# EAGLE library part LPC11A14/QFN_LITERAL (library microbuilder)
LPC11A14/QFN33 - 50MHz ARM Cortex M0 with 32kb Flash, 8kb SRAM, 10-bit ADC and DAC, Temperature Sensor, Analog Comparator, and 4kb EEPROM Temp Range: -40°C - 85°C VDD: 2.6-3.6V
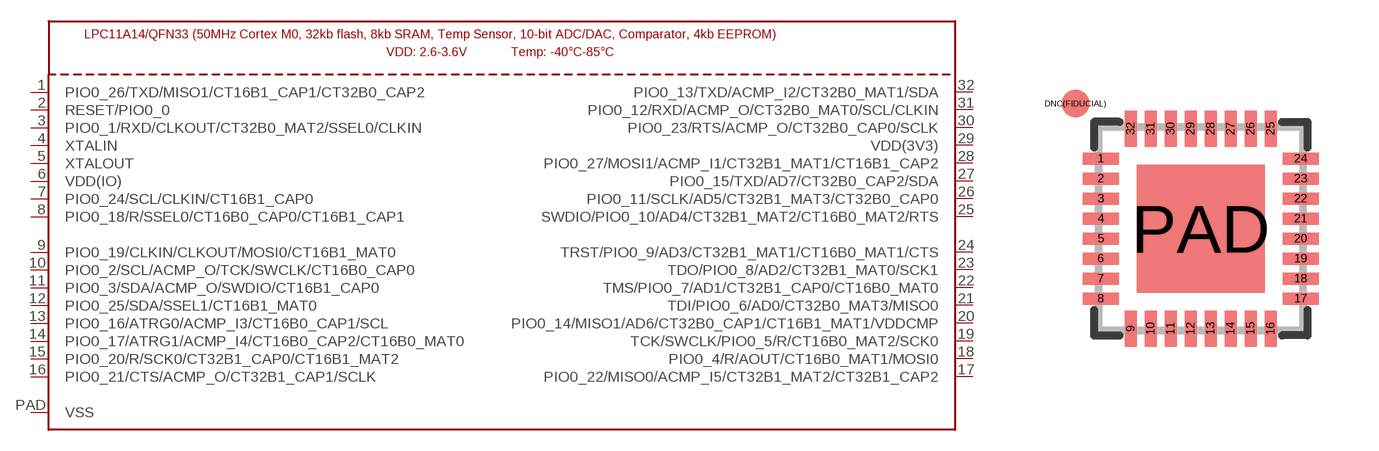
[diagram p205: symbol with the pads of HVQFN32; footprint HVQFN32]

Designator prefix U

## LPC11A14/QFN_LITERAL  [HVQFN32]
1  PIO0_26/TXD/MISO1/CT16B1_CAP1/CT32B0_CAP2
2  RESET/PIO0_0
3  PIO0_1/RXD/CLKOUT/CT32B0_MAT2/SSEL0/CLKIN
4  XTALIN  in
5  XTALOUT  out
6  VDD(IO)  sup
7  PIO0_24/SCL/CLKIN/CT16B1_CAP0
8  PIO0_18/R/SSEL0/CT16B0_CAP0/CT16B1_CAP1
9  PIO0_19/CLKIN/CLKOUT/MOSI0/CT16B1_MAT0
10  PIO0_2/SCL/ACMP_O/TCK/SWCLK/CT16B0_CAP0
11  PIO0_3/SDA/ACMP_O/SWDIO/CT16B1_CAP0
12  PIO0_25/SDA/SSEL1/CT16B1_MAT0
13  PIO0_16/ATRG0/ACMP_I3/CT16B0_CAP1/SCL
14  PIO0_17/ATRG1/ACMP_I4/CT16B0_CAP2/CT16B0_MAT0
15  PIO0_20/R/SCK0/CT32B1_CAP0/CT16B1_MAT2
16  PIO0_21/CTS/ACMP_O/CT32B1_CAP1/SCLK
17  PIO0_22/MISO0/ACMP_I5/CT32B1_MAT2/CT32B1_CAP2
18  PIO0_4/R/AOUT/CT16B0_MAT1/MOSI0
19  TCK/SWCLK/PIO0_5/R/CT16B0_MAT2/SCK0
20  PIO0_14/MISO1/AD6/CT32B0_CAP1/CT16B1_MAT1/VDDCMP
21  TDI/PIO0_6/AD0/CT32B0_MAT3/MISO0
22  TMS/PIO0_7/AD1/CT32B1_CAP0/CT16B0_MAT0
23  TDO/PIO0_8/AD2/CT32B1_MAT0/SCK1
24  TRST/PIO0_9/AD3/CT32B1_MAT1/CT16B0_MAT1/CTS
25  SWDIO/PIO0_10/AD4/CT32B1_MAT2/CT16B0_MAT2/RTS
26  PIO0_11/SCLK/AD5/CT32B1_MAT3/CT32B0_CAP0
27  PIO0_15/TXD/AD7/CT32B0_CAP2/SDA
28  PIO0_27/MOSI1/ACMP_I1/CT32B1_MAT1/CT16B1_CAP2
29  VDD(3V3)  sup
30  PIO0_23/RTS/ACMP_O/CT32B0_CAP0/SCLK
31  PIO0_12/RXD/ACMP_O/CT32B0_MAT0/SCL/CLKIN
32  PIO0_13/TXD/ACMP_I2/CT32B0_MAT1/SDA
PAD  VSS  sup

## Footprint HVQFN32 (pad centres in mm)
HVQFN32 SOT617-1 JEDEC MO-220
smd 0.9 x 0.3: 1 -2.5,1.75; 2 -2.5,1.25; 3 -2.5,0.75; 4 -2.5,0.25; 5 -2.5,-0.25; 6 -2.5,-0.75; 7 -2.5,-1.25; 8 -2.5,-1.75; 17 2.5,-1.75; 18 2.5,-1.25; 19 2.5,-0.75; 20 2.5,-0.25; 21 2.5,0.25; 22 2.5,0.75; 23 2.5,1.25; 24 2.5,1.75
smd 0.3 x 0.9: 9 -1.75,-2.5; 10 -1.25,-2.5; 11 -0.75,-2.5; 12 -0.25,-2.5; 13 0.25,-2.5; 14 0.75,-2.5; 15 1.25,-2.5; 16 1.75,-2.5; 25 1.75,2.5; 26 1.25,2.5; 27 0.75,2.5; 28 0.25,2.5; 29 -0.25,2.5; 30 -0.75,2.5; 31 -1.25,2.5; 32 -1.75,2.5
smd 0.7 x 0.7: DNC(FIDUCIAL) -3.127,3.127
smd 3.2 x 3.2: PAD 0,0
